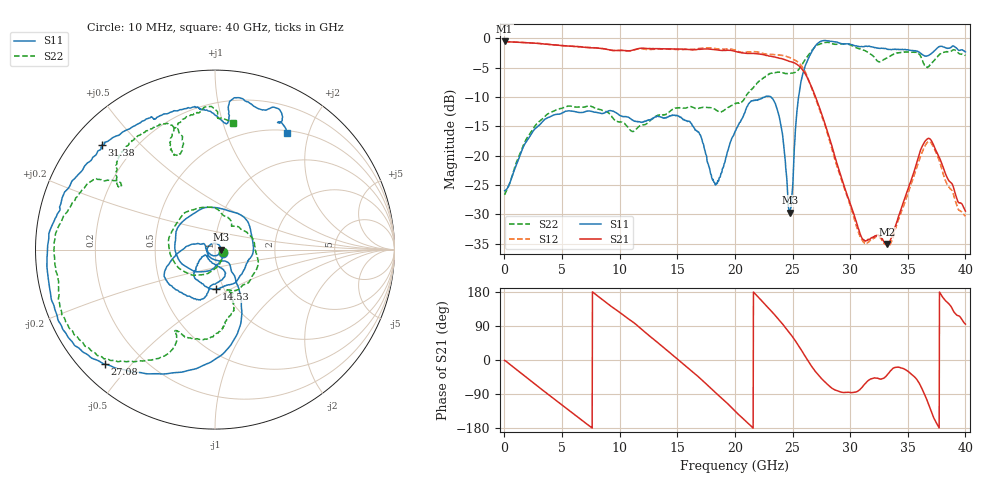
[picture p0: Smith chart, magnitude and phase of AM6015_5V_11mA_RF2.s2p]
!Agilent Technologies,E8364B,MY43040894,A.07.50.67
!Agilent E8364B: A.07.50.67
!Date: Wednesday, May 01, 2019 08:14:49
!Correction: S11(Full 2 Port(1,2))
!S21(Full 2 Port(1,2))
!S12(Full 2 Port(1,2))
!S22(Full 2 Port(1,2))
!S2P File: Measurements: S11, S21, S12, S22:
# Hz S  dB  R 50
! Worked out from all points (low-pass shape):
!   1601 points, 10 MHz to 40 GHz, reference 50 ohm
!   highest |S21| = -0.51 dB at 10 MHz (marker M1); lowest = -35.1 dB at 33.18 GHz (marker M2)
!   |S21| within 3 dB of the highest: start of sweep to 24.1 GHz
!   lowest |S11| = -29.7 dB at 24.75 GHz (marker M3), VSWR 1.07, Z = 53.4 - j0.00157 ohm
!   |S11| at or under -10 dB: start of sweep to 22.6 GHz; 23.12 GHz to 25.53 GHz (2.401 GHz wide, 9.87 % of centre)
!   |S22| runs from -26.7 to -0.7 dB; largest |S21 - S12| = 0.059
!   S11 on the Smith chart (normalised r, x): 10 MHz: 1.10, -0.04; 14.53 GHz: 0.92, -0.43; 27.08 GHz: 0.07, -0.42; 31.38 GHz: 0.09, +0.39; 40 GHz: 0.53, +1.66
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1e7  -25.97 -19.8  -0.51 -1.1  -0.51 -2.0  -26.66 -13.6
3.359162e9  -14.08 -155.0  -0.95 -80.6  -0.96 -80.6  -13.56 -144.1
6.683331e9  -12.66 120.0  -1.48 -158.4  -1.46 -158.3  -11.72 145.8
1.035741e10  -13.36 10.8  -2.08 117.1  -2.10 117.0  -14.48 64.7
1.335666e10  -13.32 -60.9  -1.78 44.4  -1.85 45.0  -13.10 13.2
1.453137e10  -13.10 -88.7  -1.81 14.6  -1.88 15.2  -12.18 -13.3
1.778056e10  -22.07 -151.1  -1.84 -71.2  -1.62 -69.9  -11.81 -61.4
1.848038e10  -24.66 -137.2  -1.96 -90.8  -1.78 -90.2  -12.36 -70.1
2.0005e10  -15.92 -70.3  -2.20 -134.7  -1.99 -134.9  -11.11 -69.3
2.170458e10  -10.59 -111.1  -2.60 176.3  -2.27 176.2  -8.21 -79.5
2.327918e10  -10.32 -156.7  -3.13 124.9  -2.75 125.7  -5.88 -100.0
2.405399e10  -15.58 175.7  -3.47 97.9  -2.89 97.5  -5.83 -110.0
2.475381e10  -29.69 -0.0  -3.95 71.2  -3.29 68.8  -5.99 -115.8
2.557861e10  -9.24 -64.8  -4.73 35.1  -4.27 30.9  -5.21 -112.9
2.667833e10  -2.26 -116.2  -8.43 -17.8  -8.59 -23.6  -2.06 -127.9
2.707823e10  -1.06 -133.9  -10.41 -33.9  -10.72 -37.9  -1.24 -135.4
2.850288e10  -0.56 -176.1  -18.95 -75.9  -19.50 -79.0  -0.95 -166.4
3.137716e10  -1.34 137.2  -34.51 -59.8  -34.92 -60.0  -2.20 149.8
3.317671e10  -1.83 115.3  -35.05 -41.0  -35.23 -41.7  -3.37 143.8
3.335166e10  -1.90 115.0  -34.87 -34.5  -35.42 -35.4  -3.13 141.9
3.677581e10  -2.93 84.3  -17.05 -114.7  -17.63 -113.2  -4.83 113.1
4e10  -2.32 58.4  -29.45 94.7  -30.34 94.9  -2.93 82.0
